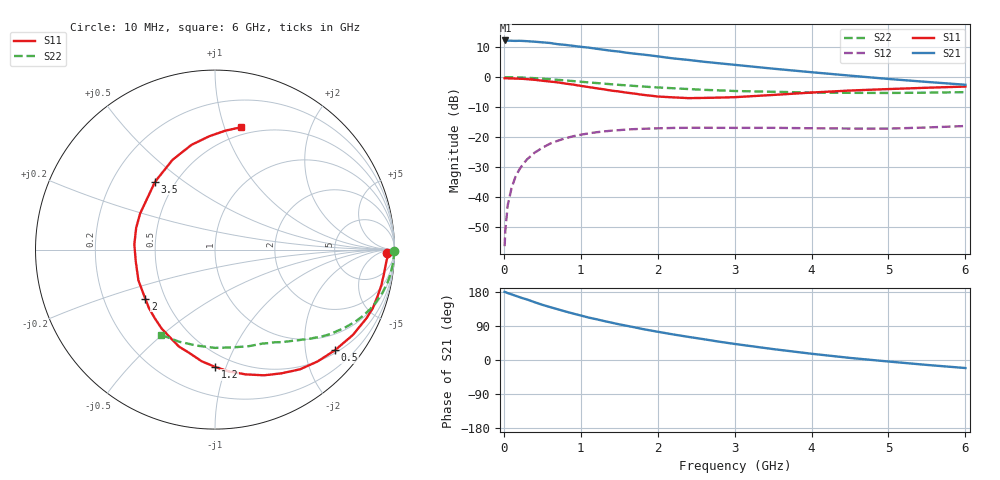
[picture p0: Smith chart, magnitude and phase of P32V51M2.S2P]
! SIEMENS Small Signal Semiconductors
! BFP181
! Si NPN RF Bipolar Junction Transistor in SOT143
! VCE = 2.5 V  IC = 1.2 mA
! Common Emitter S-Parameters:  March  1996
# GHz  S  MA  R  50
!  f  S11  S21  S12  S22
! GHz  MAG  ANG  MAG  ANG  MAG  ANG  MAG  ANG
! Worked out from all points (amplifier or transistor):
!   36 points, 10 MHz to 6 GHz, reference 50 ohm
!   highest |S21| = 12.3 dB at 20 MHz (marker M1)
!   |S21| within 3 dB of that: start of sweep to 1.269 GHz
!   unconditionally stable (mu >= 1): 2.889 GHz to end of sweep
!   at 250 MHz: K = 0.09, MSG = 20.6 dB, |S12| = -29.0 dB
!   at 1.4 GHz: K = 0.53, MSG = 13.3 dB, |S12| = -17.9 dB
!   at 6 GHz: K = 1.25, MAG = 3.9 dB, |S12| = -16.3 dB
!   S11 on the Smith chart (normalised r, x): 10 MHz: 40, -16; 500 MHz: 0.56, -2.64; 1.2 GHz: 0.40, -0.92; 2 GHz: 0.39, -0.27; 3.5 GHz: 0.39, +0.39; 6 GHz: 0.43, +1.14
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0.01  0.9574 -1.0  4.1 179.6  0.0015 78.5  0.9985 -0.3
0.02  0.965 -1.7  4.107 179.2  0.0028 91.8  0.9975 -0.7
0.05  0.9572 -3.9  4.082 176.6  0.0072 88.7  0.9967 -1.9
0.1  0.9512 -8.0  4.058 173.2  0.014 83.0  0.9959 -3.8
0.15  0.9477 -12.3  4.038 169.7  0.0215 82.3  0.9917 -5.5
0.25  0.9376 -20.4  4.028 162.7  0.0353 77.5  0.9833 -9.3
0.3  0.927 -24.3  3.994 159.9  0.0421 74.2  0.9776 -11.1
0.4  0.9033 -31.8  3.916 152.5  0.0548 69.5  0.9631 -14.5
0.5  0.8723 -40.0  3.82 145.7  0.0659 64.6  0.9449 -17.9
0.6  0.8455 -47.5  3.729 139.7  0.0775 60.0  0.9253 -21.1
0.8  0.7824 -61.8  3.462 128.1  0.0952 51.7  0.8823 -26.7
1.1  0.6835 -83.4  3.122 112.1  0.1151 40.8  0.8174 -33.7
1.2  0.6543 -89.8  2.988 107.7  0.12 37.4  0.799 -36.0
1.5  0.5761 -110.5  2.676 94.1  0.1303 29.7  0.743 -41.3
1.8  0.5079 -131.6  2.393 81.9  0.1371 23.9  0.6993 -45.8
2  0.4752 -144.9  2.227 74.6  0.1396 20.4  0.6737 -48.7
2.2  0.4598 -158.1  2.059 67.5  0.1418 17.0  0.6532 -51.6
2.8  0.4556 164.7  1.705 48.3  0.1424 10.1  0.6015 -60.0
3.5  0.5046 131.4  1.387 28.8  0.1424 5.2  0.5701 -70.7
4.5  0.5983 102.6  1.061 5.5  0.1386 2.1  0.5475 -90.1
5.5  0.6658 84.9  0.833 -13.0  0.1444 4.2  0.5509 -111.4
6  0.6966 78.0  0.747 -21.2  0.1527 4.0  0.5622 -122.4
